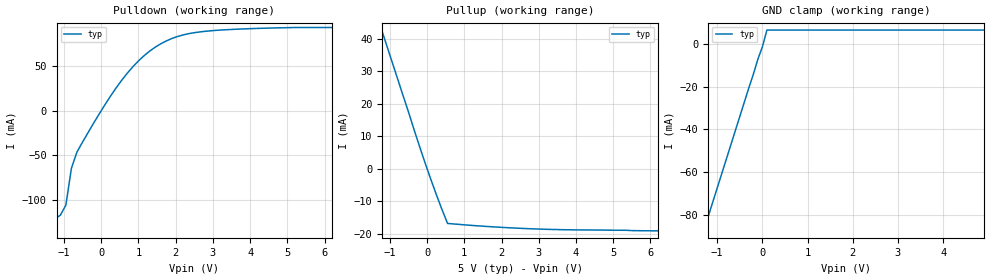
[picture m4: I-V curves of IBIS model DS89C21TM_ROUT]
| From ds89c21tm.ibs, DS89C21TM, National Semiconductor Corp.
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|   Receiver Output  MODEL
[Model]   DS89C21TM_ROUT
Model_type   Output
| Signals   ROUT
Vmeas = 2V
Cref = 50pF
Vref = 0
| variable   typ   min   max
C_comp   3.0pF   NA   NA
|   typ   min   max
[Temperature Range]   25.0   NA   NA
[Voltage range]   5.0V   4.5V   5.5V
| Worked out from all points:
|   slope of the pulldown table from 0 to 0.75 V, typ, clamps not added: 17 ohm
|   slope of the pullup table from 0 to 0.75 V, typ, clamps not added: 43.9 ohm
[Pulldown]
|   Voltage   I(typ)   I(min)   I(max)
-5V       -500mA     NA         NA
-1.4V     -135.8mA   NA         NA
-1.25V    -120.6mA   NA         NA
-1.1V     -116.7mA   NA         NA
-950mV    -105.4mA   NA         NA
-800mV    -64.29mA   NA         NA
-650mV    -46.03mA   NA         NA
100mV     6.57mA     NA         NA
1V        55.38mA    NA         NA
1.9V      80.41mA    NA         NA
4V        91.34mA    NA         NA
9.85V     92.64mA    NA         NA
[Pullup]
|   Voltage   I(typ)   I(min)   I(max)
| Note that the[Pullup]voltage table is referenced to Vcc
| and is calculated using Vtable=Vcc - Vmeasured.
-4.85V    170.2mA    NA         NA
-1.25V    43.77mA    NA         NA
-1.1V     38.5mA     NA         NA
-50mV     1.71mA     NA         NA
250mV     -7.947mA   NA         NA
550mV     -16.79mA   NA         NA
1.9V      -17.94mA   NA         NA
3.25V     -18.62mA   NA         NA
10V       -19.69mA   NA         NA
[GND_clamp]
|   Voltage   I(typ)   I(min)   I(max)
-5V       -336.3mA   NA         NA
-1.3V     -87.62mA   NA         NA
-200mV    -14mA      NA         NA
-100mV    -6.957mA   NA         NA
0V        -1.15mA    NA         NA
100mV     6.722mA    NA         NA
4.9V      6.722mA    NA         NA
[POWER_clamp]
|   Voltage   I(typ)   I(min)   I(max)
| Note that the[POWER_clamp]voltage table is referenced to Vcc
| and is calculated using Vtable=Vcc - Vmeasured.
5.05V     0A         NA         NA
5.1V      0A         NA         NA
5.15V     0A         NA         NA
10V       0A         NA         NA
[Ramp]
|   typ   min   max
dV/dt_r   2.88/2.5n   NA   NA
dV/dt_f   2.88/2.1n   NA   NA
R_load = 1MOhm
